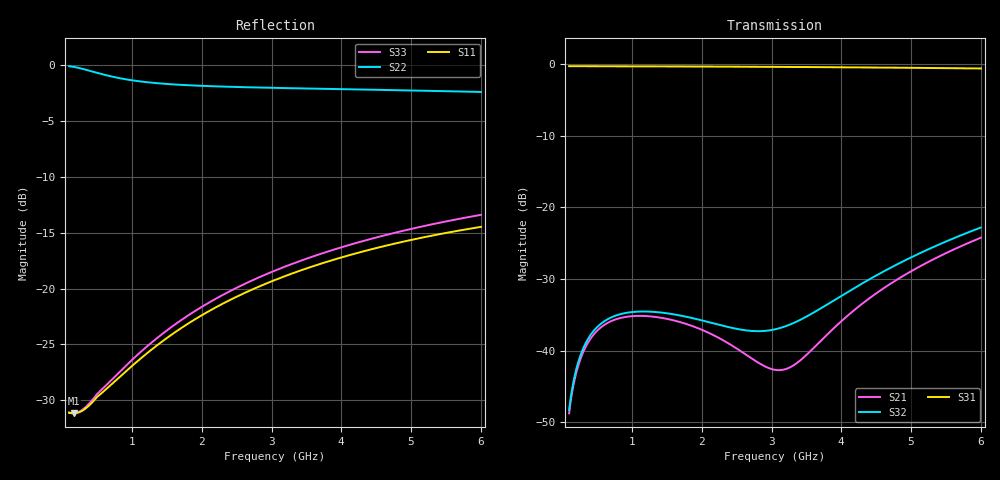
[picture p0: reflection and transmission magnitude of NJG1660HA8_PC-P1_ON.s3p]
! NJG1660HA8 S-parameter(touchstone)
! 2bit SPDT switch
! Port1=P1, Port2=P2, Port3=PC
! VCTL(H)=3.0V, VCTL(L)=0.0V, PC-P1 ON
!  /-o P1(Port1)
!  PC  o-
! (Port3)  -o P2(Port2)
# hz S ma R 50
! 3 Port Network Data from SP1.SP block
! freq  magS11  angS11  magS12  angS12  magS13  angS13
!  magS21  angS21
!  magS22  angS22  magS23  angS23
!  magS31  angS31  magS32  angS32
!  magS33  angS33
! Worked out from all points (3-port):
!   591 points, 100 MHz to 6 GHz, reference 50 ohm
!   strongest paths, dB at 100 MHz, 1.57 GHz, 3.05 GHz, 4.53 GHz, 6 GHz:
!     S31: -0.3, -0.3, -0.4, -0.5, -0.6
!     S32: -48.2, -34.9, -37.0, -29.3, -22.8
!     S21: -48.7, -35.7, -42.7, -31.8, -24.2
!   lowest |S11| = -31.2 dB at 170 MHz (marker M1), VSWR 1.06, Z = 52.8 - j0.248 ohm
!   |S11| at or under -10 dB: start of sweep to end of sweep
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1e8  0.02783 3.7  0.003663 71.1  0.9676 -1.6
     0.003662 71.1  0.9903 -17.0  0.003868 72.9
     0.9676 -1.6  0.003869 72.9  0.02779 3.1
1.7e8  0.02761 -4.9  0.006002 67.1  0.9674 -2.0
       0.006001 67.1  0.9828 -28.3  0.006357 69.2
       0.9674 -2.0  0.006357 69.2  0.02764 -5.8
3.5e8  0.02924 -25.5  0.01094 54.9  0.9669 -3.2
       0.01094 54.9  0.9527 -54.9  0.01161 57.8
       0.9669 -3.2  0.01161 57.8  0.02972 -26.9
5.4e8  0.03347 -42.2  0.01436 44.3  0.9663 -4.5
       0.01436 44.3  0.9176 -78.3  0.01521 48.2
       0.9663 -4.5  0.01521 48.2  0.0346 -43.3
8.4e8  0.04059 -57.3  0.01696 31.1  0.9655 -6.9
       0.01696 31.1  0.8729 -106.5  0.01804 37.3
       0.9655 -6.9  0.01804 37.3  0.04286 -57.6
1.19e9  0.0505 -70.0  0.01748 21.1  0.9647 -9.8
        0.01748 21.1  0.8411 -129.4  0.01879 30.4
        0.9647 -9.8  0.01879 30.4  0.05416 -69.0
1.92e9  0.07331 -87.6  0.01454 12.0  0.9623 -15.8
        0.01454 12.0  0.8104 -159.4  0.01667 29.3
        0.9623 -15.8  0.01667 29.3  0.07986 -83.7
3.05e9  0.1092 -106.0  0.007361 48.6  0.957 -25.0
        0.007361 48.6  0.7916 172.2  0.01411 65.5
        0.957 -25.0  0.01411 65.5  0.1203 -97.8
4.71e9  0.1574 -127.5  0.02947 107.5  0.9451 -38.7
        0.02947 107.5  0.774 141.5  0.03804 103.5
        0.9451 -38.7  0.03804 103.5  0.1759 -112.8
6e9  0.1888 -143.3  0.06152 97.7  0.9324 -49.3
     0.06153 97.7  0.7591 119.5  0.07247 100.3
     0.9324 -49.3  0.07247 100.3  0.2138 -122.8
